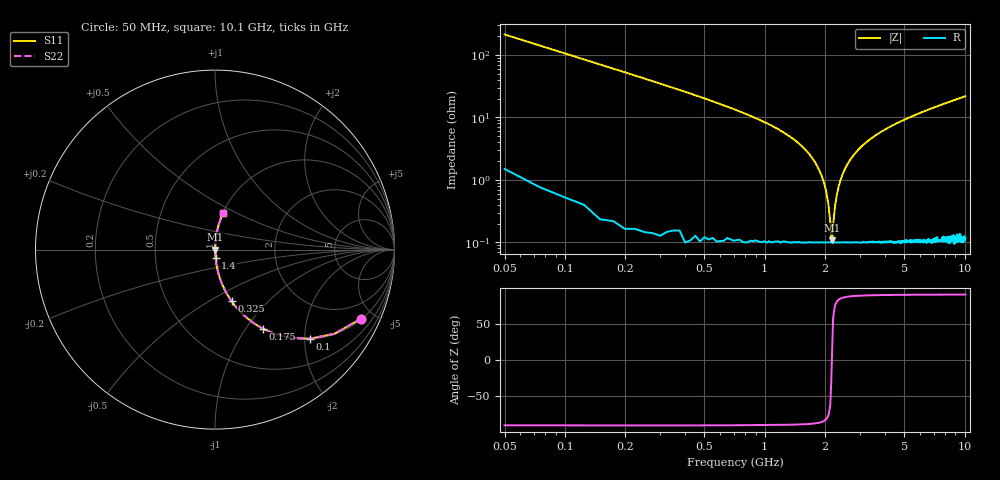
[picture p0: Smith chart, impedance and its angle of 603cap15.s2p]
! AVX Thin Film Operation		Date: November 2004
! Description: Accu-P® Series, Thin Film, SMD, RF Capacitor
! Part Number: 06033J150FBT
! 50 MHz  -  10.05 GHz
! Serial Measurements
# hz S db R 50
!	S11		S21		S12		S22
!	dB	Phase	dB	Phase	dB	Phase	dB	Phase
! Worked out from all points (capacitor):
!   400 points, 50 MHz to 10.1 GHz, reference 50 ohm
!   read as one part in series: C = 15 pF near 100 MHz
!   lowest |Z| = 108 mohm at 2.18 GHz (marker M1)
!   series resonance near 2.169 GHz, so ESL is about 360 pH
!   S11 on the Smith chart (normalised r, x): 50 MHz: 1.03, -4.24; 100 MHz: 1.01, -2.12; 175 MHz: 1.00, -1.20; 325 MHz: 1.00, -0.63; 1.4 GHz: 1.00, -0.09; 10.1 GHz: 1.00, +0.43
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5e7  -0.90 -25.2  -7.43 64.4  -7.43 64.4  -0.90 -25.2
1e8  -2.79 -43.2  -3.28 46.5  -3.28 46.5  -2.79 -43.2
1.75e8  -5.76 -58.8  -1.36 31.0  -1.36 31.0  -5.76 -58.8
3.25e8  -10.40 -72.1  -0.43 17.7  -0.43 17.7  -10.40 -72.1
7e8  -17.40 -81.8  -0.09 7.7  -0.09 7.7  -17.40 -81.8
1.4e9  -27.10 -86.2  -0.02 2.5  -0.02 2.5  -27.10 -86.2
1.73e9  -33.00 -86.2  -0.01 1.3  -0.01 1.3  -33.00 -86.2
2.03e9  -43.50 -81.0  -0.01 0.4  -0.01 0.4  -43.50 -81.0
2.08e9  -47.30 -76.4  -0.01 0.2  -0.01 0.2  -47.30 -76.4
2.13e9  -53.50 -61.7  -0.01 0.1  -0.01 0.1  -53.50 -61.7
2.15e9  -58.20 -35.7  -0.01 0.0  -0.01 0.0  -58.20 -35.7
2.18e9  -59.30 22.5  -0.01 -0.0  -0.01 -0.0  -59.30 22.5
2.2e9  -54.80 56.8  -0.01 -0.1  -0.01 -0.1  -54.80 56.8
2.25e9  -48.30 74.8  -0.01 -0.2  -0.01 -0.2  -48.30 74.8
2.35e9  -41.90 82.4  -0.01 -0.5  -0.01 -0.5  -41.90 82.4
2.45e9  -38.30 84.6  -0.01 -0.7  -0.01 -0.7  -38.30 84.6
2.75e9  -32.50 86.2  -0.01 -1.4  -0.01 -1.4  -32.50 86.2
3.4e9  -26.80 86.1  -0.02 -2.6  -0.02 -2.6  -26.80 86.1
5.08e9  -20.60 84.0  -0.05 -5.4  -0.05 -5.4  -20.60 84.0
6.75e9  -17.40 81.8  -0.09 -7.8  -0.09 -7.8  -17.40 81.8
8.43e9  -15.10 79.6  -0.14 -10.1  -0.14 -10.1  -15.10 79.6
1.01e10  -13.50 77.5  -0.21 -12.2  -0.21 -12.2  -13.50 77.5
